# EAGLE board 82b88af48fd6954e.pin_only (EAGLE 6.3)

Size 19.05 x 17.78 mm. Coordinates in mm from the lower left corner, seen from the top.
Outline: 19.05,15.24 19.05,2.54 arc-90 16.51,0 2.54,0 arc-90 0,2.54 0,15.24 arc-90 2.54,17.78 16.51,17.78 arc-90 19.05,15.24
Copper layers (1*16): Top 0.035mm / dielectric 1.5mm / Bottom 0.035mm
Design rules "adafruit": minimum track width 8mil, minimum drill 15.5mil, track to track 8mil, track to pad 8mil, pad to pad 8mil, via to via 8mil, smd to smd 8mil, copper to edge 10mil, drill to drill 8mil, minimum pad ring 10mil, minimum via ring 8mil, stop-mask expansion 2mil, vias tented up to drill 20mil, thermal gap 10mil

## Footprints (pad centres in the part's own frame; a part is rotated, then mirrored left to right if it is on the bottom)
0805-NO = smd 1.3 x 1.5: 1 -0.95,0; 2 0.95,0
FIDUCIAL_1MM = smd 1 x 1: 1 0,0
LGA8 = smd 1.9 x 0.6: P$1 -1.5,1.875; P$2 -1.5,0.625; P$3 -1.5,-0.625; P$4 -1.5,-1.875; P$5 1.5,-1.875; P$6 1.5,-0.625; P$7 1.5,0.625; P$8 1.5,1.875
1X07_ROUND_70 = drill 1 pad 1.778 square: 1 -7.62,0 | drill 1 pad 1.778: 2 -5.08,0; 3 -2.54,0; 4 0,0; 5 2.54,0; 6 5.08,0; 7 7.62,0
SOT23-WIDE = smd 1 x 1.2: 1 -0.95,-1; 2 0.95,-1; 3 0,1
SOT23-5 = smd 0.55 x 1.2: 1 -0.95,-1.3; 2 0,-1.3; 3 0.95,-1.3; 4 0.95,1.3; 5 -0.95,1.3
MOUNTINGHOLE_2.5_PLATED = drill 2.5 pad 3.2: P$1 0,0

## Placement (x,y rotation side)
C1  0.1µF  [0805-NO]  5.62,6.4 270 top
C2  0.1µF  [0805-NO]  2.67,11.68 0 top
C3  10uF  [0805-NO]  2.79,5.59 0 top
C4  10uF  [0805-NO]  5.59,10.03 270 top
FID1  FIDUCIAL""  [FIDUCIAL_1MM]  14.93,4.5 0 top
FID2  FIDUCIAL""  [FIDUCIAL_1MM]  5.43,16.61 0 top
IC1  MPL3115A2LGA  [LGA8]  9.78,8.38 0 top
JP2  [1X07_ROUND_70]  9.53,2.54 0 top
Q1  BSS138  [SOT23-WIDE]  14.61,10.92 180 top
Q2  BSS138  [SOT23-WIDE]  14.61,7.24 180 top
R3  10K  [0805-NO]  17.4,10.92 270 top
R4  10K  [0805-NO]  17.4,7.11 270 top
R5  10K  [0805-NO]  7.24,12.7 0 top
R6  10K  [0805-NO]  10.92,12.57 180 top
U2  MIC5225-3.3  [SOT23-5]  2.67,8.64 0 top
U$8  MOUNTINGHOLE2.5  [MOUNTINGHOLE_2.5_PLATED]  2.54,15.24 0 top
U$9  MOUNTINGHOLE2.5  [MOUNTINGHOLE_2.5_PLATED]  16.51,15.24 0 top
U$14  [ADAFRUIT_3.5MM]  10.8,13.57 0 bottom

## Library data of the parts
C1-C4 IC1 JP2 Q1 Q2 R3-R6 U2 U$14 = microbuilder
FID1 FID2 U$8 U$9 = microbuilder; BOM: EXCLUDE

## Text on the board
tPlace: Altimeter | MPL3115A2 | Vin | 3vo | INT1 | SDA | GND | INT2 | SCL
bPlace: I2C Barometric | Pressure & / Altimeter & / Temperature | Vin&Logic:2.5-5V | adafruit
